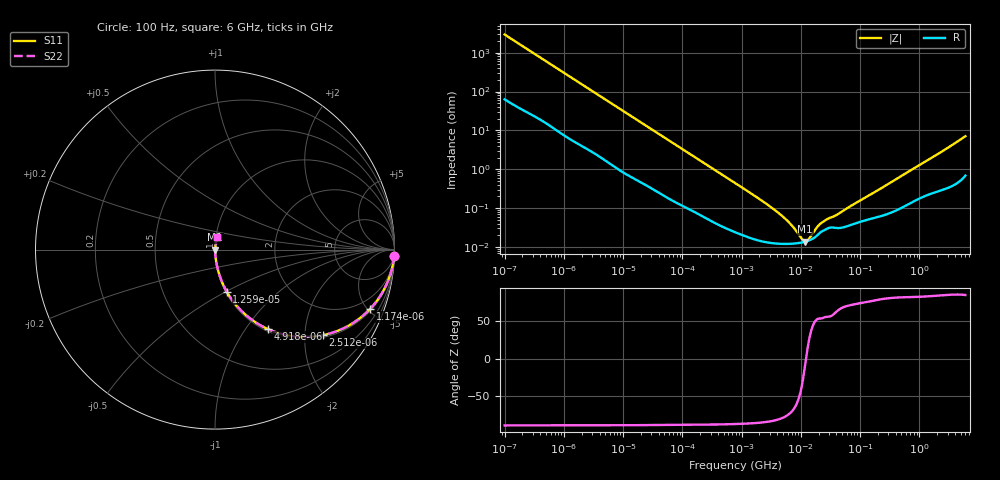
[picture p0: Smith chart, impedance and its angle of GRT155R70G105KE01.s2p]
!Murata Part Number: GRT155R70G105KE01
!These Parameters are Measured in Series Mode Connection
!Data Generated on Jun 19, 2026
!  o--ll--o
!Port1  Port2
!  o------o
!Operation Temp=25[degC], DC Bias Voltage=0[V]
!Freq. Start=100[Hz] Stop=6[GHz] 401[Steps]
# Hz S RI R 50
!Freq.(Hz) S11(Real) S11(Imag) S21(Real) S21(Imag) S12(Real) S12(Imag) S22(Real) S22(Imag)
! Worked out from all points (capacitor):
!   401 points, 100 Hz to 6 GHz, reference 50 ohm
!   read as one part in series: C = 539 nF near 109 Hz
!   lowest |Z| = 13.8 mohm at 11.89 MHz (marker M1)
!   series resonance near 12.26 MHz, so ESL is about 310 pH
!   S11 on the Smith chart (normalised r, x): 100 Hz: 2, -59; 1.174 kHz: 1.13, -5.20; 2.512 kHz: 1.07, -2.46; 4.918 kHz: 1.03, -1.27; 12.59 kHz: 1.01, -0.50; 6 GHz: 1.01, +0.14
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100  0.9981 -0.0339  0.00188 0.0339  0.00188 0.0339  0.9981 -0.0339
401  0.9793 -0.1303  0.0207 0.1303  0.0207 0.1303  0.9793 -0.1303
750  0.9373 -0.2303  0.0627 0.2303  0.0627 0.2303  0.9373 -0.2303
1174  0.8652 -0.3294  0.1348 0.3294  0.1348 0.3294  0.8652 -0.3294
2008  0.6966 -0.447  0.3034 0.447  0.3034 0.447  0.6966 -0.447
2512  0.5993 -0.4769  0.4007 0.4769  0.4007 0.4769  0.5993 -0.4769
4918  0.2931 -0.442  0.7069 0.442  0.7069 0.442  0.2931 -0.442
7695  0.15 -0.3442  0.85 0.3442  0.85 0.3442  0.15 -0.3442
12592  0.0652 -0.2339  0.9348 0.2339  0.9348 0.2339  0.0652 -0.2339
40335  0.00882 -0.0794  0.9912 0.0794  0.9912 0.0794  0.00882 -0.0794
774597  0.00026 -0.00443  0.9997 0.00443  0.9997 0.00443  0.00026 -0.00443
4440638  0.000121 -0.000692  0.9999 0.000692  0.9999 0.000692  0.000121 -0.000692
6948629  0.000121 -0.000346  0.9999 0.000346  0.9999 0.000346  0.000121 -0.000346
1.039699e7  0.000131 -9.59e-05  0.9999 9.59e-05  0.9999 9.59e-05  0.000131 -9.59e-05
1.189169e7  0.000137 -1.75e-05  0.9999 1.75e-05  0.9999 1.75e-05  0.000137 -1.75e-05
1.360128e7  0.000146 6.08e-05  0.9999 -6.08e-05  0.9999 -6.08e-05  0.000146 6.08e-05
1.555665e7  0.00016 0.00014  0.9998 -0.00014  0.9998 -0.00014  0.00016 0.00014
2.035112e7  0.000222 0.000297  0.9998 -0.000297  0.9998 -0.000297  0.000222 0.000297
2.545746e7  0.000274 0.000391  0.9997 -0.000391  0.9997 -0.000391  0.000274 0.000391
4.165952e7  0.000307 0.000617  0.9997 -0.000617  0.9997 -0.000617  0.000307 0.000617
3.124326e8  0.000752 0.00428  0.9992 -0.00428  0.9992 -0.00428  0.000752 0.00428
6e9  0.0117 0.0692  0.9883 -0.0692  0.9883 -0.0692  0.0117 0.0692
